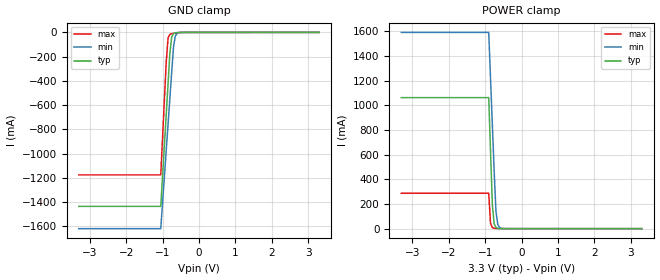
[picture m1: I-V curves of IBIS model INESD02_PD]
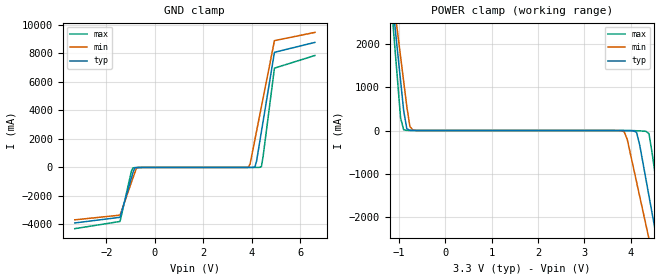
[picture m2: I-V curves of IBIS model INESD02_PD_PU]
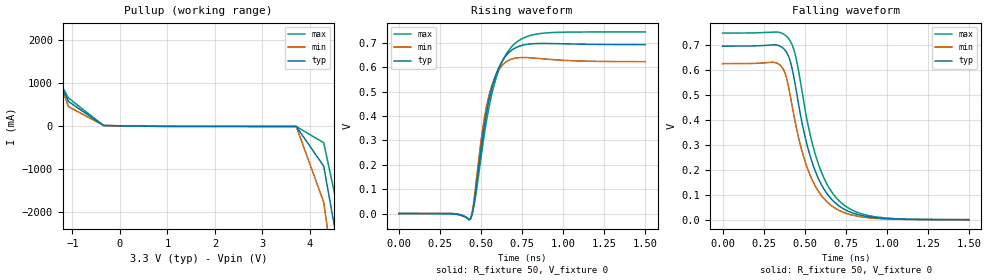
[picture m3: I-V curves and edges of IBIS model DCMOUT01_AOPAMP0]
|   This file is an IBIS representation of the   |
|   Integrated Device Technology , Inc.   |
|   ICS9DB202-01   |
|   PCI Express Jitter Attenuator   |
[IBIS Ver]   4.1
[File name]   9db202_01_3v3.ibs
[File Rev]   2.0
[Date]   27 Aug 2009 | Last modified
|   Jul 01 2003 | Generated
[Source]   Originated at Integrated Device Technology, Inc.
[Disclaimer]
IDT hereby grants the user of this IBIS model a non-exclusive,
nontransferable license to use this IBIS model under the following terms.
Before using this IBIS model, the user should read this license.
If the user does not accept these terms,  the IBIS model should be
returned to IDT within 30 days.
   The user is granted this license only to use the IBIS model and
is not granted rights to sell, load, rent, lease or license the IBIS
model in whole or in part, or in modified form to anyone other than
user. User may modify the IBIS model to suit its specific
applications but rights to derivative works and such modifications
shall belong to IDT.
   This IBIS model is provided on an "AS IS" basis and IDT makes
absolutely no warranty with respect to the information contained
herein. IDT DISCLAIMS AND CUSTOMER WAIVES ALL WARRANTIES, EXPRESS
OR IMPLIED, INCLUDING WARRANTIES OF MERCHANTABILITY OR FITNESS FOR
A PARTICULAR PURPOSE. The entire risk as to quality and performance
is with the Customer. ACCORDINGLY, IN NO EVENT SHALL THE COMPANY BE
LIABLE FOR ANY DAMAGES, WHETHER IN CONTRACT OR TORT,INCLUDING ANY
LOST PROFITS OR OTHER INCIDENTAL, CONSEQUENTIAL, EXEMPLARY, OR
PUNITIVE DAMAGES ARISING OUT OF THE USE OR APPLICATION OF THE IBIS
model provided in this package. Further, IDT reserves the right to
make changes without notice to any product herein to improve
reliability, function, or design. IDT does not convey any license
under patent rights or any other intellectual property rights,
including those of third parties.
   IDT is not obligated to provide maintenance or support
for the licensed IBIS model.
[Copyright]   Copyright 2004 by Integrated Device Technology , Inc.
[Component]   ICS9DB202-01
[Manufacturer] Integrated Device Technology, Inc.
[Package]
|QFN32
|lead+wire  typ   min   max
R_pkg   72.4655m   58.886m   86.045m
L_pkg   1.47175nH   1.11650nH   1.77850nH
C_pkg   0.07747pF   0.07444pF   0.08050pF
[Pin]   signal_name   model_name   R_pin   L_pin   C_pin
1   IREF   NC   86.045m   1.77850nH   0.08050pF
2   NC   NC   76.996m   1.55783nH   0.07848pF
3   VDDA   POWER   67.941m   1.33717nH   0.07646pF
4   CLK   INESD02_PD   58.886m   1.11650nH   0.07444pF
5   nCLK   INESD02_PD_PU   58.886m   1.11650nH   0.07444pF
6   NC   NC   67.941m   1.33717nH   0.07646pF
7   NC   NC   76.996m   1.55783nH   0.07848pF
8   NC   NC   86.045m   1.77850nH   0.08050pF
9   PCIEXT0   DCMOUT01_AOPAMP0   86.045m   1.77850nH   0.08050pF
10   PCIEXC0   DCMOUT01_AOPAMP0   76.996m   1.55783nH   0.07848pF
11   NC   NC   67.941m   1.33717nH   0.07646pF
12   NC   NC   58.886m   1.11650nH   0.07444pF
13   VDD   POWER   58.886m   1.11650nH   0.07444pF
14   NC   NC   67.941m   1.33717nH   0.07646pF
15   NC   NC   76.996m   1.55783nH   0.07848pF
16   NC   NC   86.045m   1.77850nH   0.08050pF
17   NC   NC   86.045m   1.77850nH   0.08050pF
18   NC   NC   76.996m   1.55783nH   0.07848pF
19   NC   NC   67.941m   1.33717nH   0.07646pF
20   VDD   POWER   58.886m   1.11650nH   0.07444pF
21   NC   NC   58.886m   1.11650nH   0.07444pF
22   NC   NC   67.941m   1.33717nH   0.07646pF
23   NC   NC   76.996m   1.55783nH   0.07848pF
24   NC   NC   86.045m   1.77850nH   0.08050pF
25   NC   NC   86.045m   1.77850nH   0.08050pF
26   NC   NC   76.996m   1.55783nH   0.07848pF
27   GND   GND   67.941m   1.33717nH   0.07646pF
28   NC   NC   58.886m   1.11650nH   0.07444pF
29   NC   NC   58.886m   1.11650nH   0.07444pF
30   NC   NC   67.941m   1.33717nH   0.07646pF
31   NC   NC   76.996m   1.55783nH   0.07848pF
32   NC   NC   86.045m   1.77850nH   0.08050pF
[Diff Pin]  inv_pin  vdiff tdelay_typ tdelay_min  tdelay_max
4   5   0.15   0   0   0
9   10   NA   0   0   0
| Models and submodels in the file (3): INESD02_PD (Input), INESD02_PD_PU (Input), DCMOUT01_AOPAMP0 (Open_source)
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[Model]   INESD02_PD
Model_type   Input
Polarity   Non-Inverting
Vinl = 0.80V
Vinh = 2.0V
|   typ   min   max
C_comp   2pF   1.5pF   2.5pF
|   typ   min   max
[Voltage range]  3.3V   3.15V   3.45V
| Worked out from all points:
|   GND clamp passes 1 mA (typ) near -0.56 V on its own axis
|   POWER clamp passes 1 mA (typ) near -0.61 V on its own axis
[GND_clamp]
|Voltage   I(typ)   I(min)   I(max)
-3.3V     -1.436A    -1.62A     -1.176A
-1.05V    -1.436A    -1.62A     -1.176A
-900mV    -678.5mA   -975.1mA   -244mA
-850mV    -426.1mA   -760.1mA   -46.85mA
-800mV    -173.9mA   -545.4mA   -16.11mA
-750mV    -36.96mA   -330.7mA   -9.916mA
-700mV    -9.696mA   -120.2mA   -7.056mA
-650mV    -3.545mA   -29.7mA    -4.857mA
-600mV    -1.629mA   -7.52mA    -3.049mA
-400mV    -52.81uA   -52.52uA   -108.7uA
3.3V      71.13uA    77.43uA    62.11uA
[POWER_clamp]
|Voltage   I(typ)   I(min)   I(max)
-3.3V     1.063A     1.593A     287.3mA
-900mV    1.063A     1.593A     287.3mA
-850mV    620.5mA    1.215A     41.84mA
-800mV    191.6mA    837.5mA    8.757mA
-750mV    37.76mA    460.2mA    3.328mA
-700mV    8.104mA    133.8mA    1.728mA
-650mV    2.076mA    32.66mA    905.3uA
-600mV    678.1uA    8.083mA    443.8uA
-450mV    104.2uA    213.3uA    89.09uA
3.3V      -3.041nA   -3.986uA   0A
[Model]   INESD02_PD_PU
Model_type  Input
Polarity   Non-Inverting
Vinl = 0.8V
Vinh = 2.0V
|   typ   min   max
C_comp   2pF   1.5pF   2.5pF
|   typ   min   max
[Voltage range]   3.3V   3.15V   3.45V
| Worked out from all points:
|   GND clamp passes 1 mA (typ) near -0.59 V on its own axis
|   POWER clamp passes 1 mA (typ) near -0.70 V on its own axis
[GND_clamp]
-3.3V     -3.894A    -3.674A    -4.294A
-1.433V   -3.498A    -3.345A    -3.788A
-963.9mV  -730.3mA   -1.043A    -250mA
-896.9mV  -335.4mA   -714.8mA   -27.09mA
-695.9mV  -3.422mA   -10.72mA   -6.487mA
3.861V    132.6uA    27.79mA    76.29uA
3.928V    264.4uA    239.1mA    80.1uA
4.129V    40.53mA    1.967A     342uA
4.196V    445.9mA    2.544A     962.5uA
4.397V    2.525A     4.275A     64.09mA
4.933V    8.079A     8.897A     6.966A
6.6V      8.773A     9.475A     7.854A
[POWER_clamp]
-3.3V     6.7A       6.327A     7.39A
-1.165V   3.23A      3.44A      2.951A
-1.031V   1.843A     2.286A     1.176A
-963.9mV  1.149A     1.709A     289.6mA
-896.9mV  456.5mA    1.133A     15.41mA
-695.9mV  812.8uA    10.76mA    565.7uA
3.861V    -638.5uA   -26.24mA   -108.3uA
4.129V    -41.93mA   -1.19A     -4.977mA
4.33V     -1.119A    -2.176A    -17.94mA
4.531V    -2.305A    -3.163A    -1.019A
4.732V    -3.492A    -4.151A    -2.536A
6.6V      -5.075A    -5.469A    -4.558A
[Model]   DCMOUT01_AOPAMP0
Model_type   Open_source
Polarity   Non-Inverting
|   typ   min   max
C_comp   2pF   1.5pF   2.5pF
Vmeas = 0.313V
Rref = 50
Cref = 0
Vref = 0V
|   typ   min   max
[Voltage range]   3.3V   3.135V   3.465V
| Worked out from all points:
|   slope of the pullup table from 0 to 0.495 V, typ, clamps not added: 56.7 ohm
|   rising waveform, R_fixture 50, V_fixture 0: 20-80 % time 106ps typ, 84.7ps min, 129ps max; typ from 0 V to 0.694 V
|   falling waveform, R_fixture 50, V_fixture 0: 20-80 % time 164ps typ, 161ps min, 167ps max; typ from 0.694 V to 0 V
[Pullup]
|Voltage   I (typ)   I (min)   I (max)
-3.3V     5.929A     7.281A     5.127A
-2.56V    4.138A     4.999A     3.631A
-1.82V    2.348A     2.721A     2.135A
-1.08V    565.1mA    446mA      646.5mA
-340mV    7.043mA    7.923mA    6.433mA
3.71V     -13.96mA   -13.12mA   -14.97mA
4.288V    -938.8mA   -1.777A    -394.6mA
4.866V    -4.53A     -6.36A     -3.385A
6.6V      -15.32A    -20.11A    -12.39A
[Ramp]
|   typ   min   max
dV/dt_r   0.579/0.169n   0.532/0.14n   0.616/0.204n
dV/dt_f   0.559/0.267n   0.503/0.26n   0.6/0.273n
R_load =   50.0000
[Rising Waveform]
R_fixture = 50
V_fixture = 0   | VCC_typ
V_fixture_max = 0   | VCC_max
V_fixture_min = 0   | VCC_min
C_fixture = 0.0p
| Time   typ   min   max
0s        1.466nV    326.9pV    95.28nV
324.3ps   -487.2uV   117.6uV    -1.252mV
435.4ps   -22.14mV   -21.08mV   -20.84mV
458ps     43.19mV    59.96mV    35.8mV
512ps     324.5mV    357.6mV    289.8mV
551.1ps   474.6mV    491.9mV    445.6mV
612.6ps   606.4mV    595mV      598.3mV
690.7ps   673.1mV    635.4mV    688.5mV
876.9ps   698.5mV    635.3mV    740.5mV
1.498ns   693.8mV    623.8mV    745.7mV
[Falling Waveform]
R_fixture = 50
V_fixture = 0   | VCC_typ
V_fixture_max = 0   | VCC_max
V_fixture_min = 0   | VCC_min
C_fixture = 0.0p
| Time   typ   min   max
0s        693.6mV    623.5mV    745.6mV
328.8ps   698mV      626.2mV    750mV
403.9ps   648.3mV    522mV      721.7mV
439.9ps   546.3mV    395mV      664.6mV
477.5ps   405.9mV    287.5mV    535mV
555.6ps   208.2mV    144.4mV    280.1mV
635.1ps   103.9mV    71.07mV    141.6mV
738.7ps   42.2mV     28.35mV    58.32mV
958ps     6.335mV    4.085mV    9.051mV
1.498ns   59.76uV    34.68uV    93.36uV
